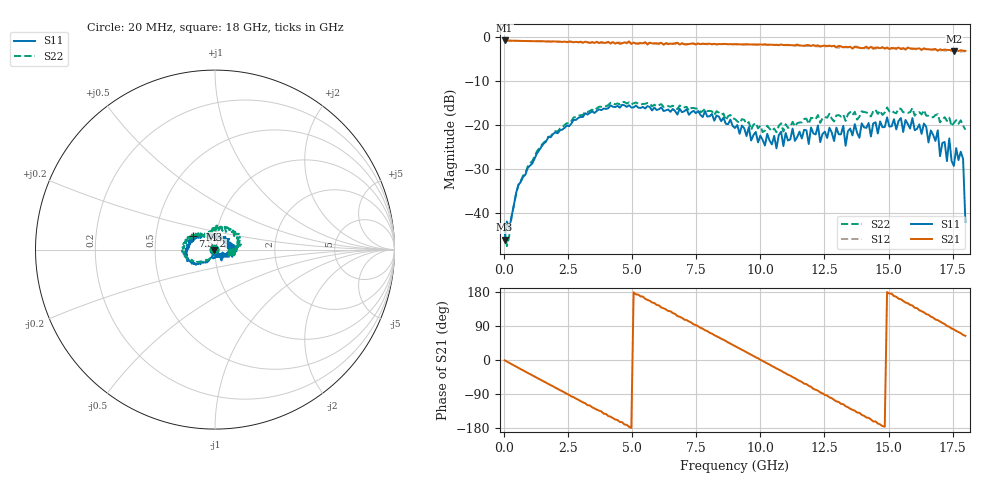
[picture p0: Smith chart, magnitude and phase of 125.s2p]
!Agilent Technologies,N5230A,US43500223,A.07.50.48
!Agilent N5230A: A.07.50.48
!Date: Sunday, January 31, 2016 17:07:24
!Correction: S11(Full 2 Port(1,2))
!S21(Full 2 Port(1,2))
!S12(Full 2 Port(1,2))
!S22(Full 2 Port(1,2))
!S2P File: Measurements: S11, S21, S12, S22:
# Hz S  RI  R 50
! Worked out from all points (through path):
!   201 points, 20 MHz to 18 GHz, reference 50 ohm
!   highest |S21| = -0.70 dB at 20 MHz (marker M1); lowest = -3.1 dB at 17.55 GHz (marker M2)
!   group delay of S21, straight-line fit = 101 ps
!   lowest |S11| = -46.1 dB at 20 MHz (marker M3), VSWR 1.01, Z = 49.5 + j0.051 ohm
!   |S11| at or under -10 dB: start of sweep to end of sweep
!   |S22| runs from -47.6 to -14.7 dB; largest |S21 - S12| = 0.07
!   S11 on the Smith chart (normalised r, x): 20 MHz: 0.99, +0.00; 7.572 GHz: 0.77, +0.12; 18 GHz: 1.00, -0.02
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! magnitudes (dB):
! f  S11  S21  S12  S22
! 20 MHz  -46.1  -0.7  -0.7  -44.0
! 109.9 MHz  -41.9  -0.7  -0.7  -47.6
! 559.4 MHz  -33.6  -0.8  -0.8  -33.6
! 1.279 GHz  -26.4  -0.9  -0.9  -26.0
! 3.077 GHz  -18.1  -1.2  -1.1  -17.7
! 6.043 GHz  -16.4  -1.4  -1.6  -15.4
! 7.572 GHz  -16.8  -1.4  -1.3  -16.2
! 9.01 GHz  -20.6  -1.5  -1.5  -18.6
! 10.63 GHz  -25.3  -1.7  -1.7  -21.6
! 12.07 GHz  -21.9  -1.7  -1.9  -18.4
! 13.24 GHz  -20.1  -2.3  -2.2  -17.6
! 13.33 GHz  -24.7  -2.1  -2.2  -19.0
! 15.03 GHz  -20.3  -2.7  -2.6  -16.9
! 16.92 GHz  -21.2  -3.0  -3.0  -17.5
! 17.01 GHz  -27.1  -2.7  -3.0  -19.3
! 17.19 GHz  -23.8  -2.8  -3.0  -18.2
! 17.28 GHz  -28.2  -2.9  -3.0  -19.0
! 17.37 GHz  -23.0  -2.9  -3.1  -18.3
! 17.55 GHz  -29.3  -3.1  -3.2  -19.5
! 17.64 GHz  -25.2  -2.9  -3.1  -18.9
! 17.91 GHz  -27.7  -3.0  -3.1  -20.1
! 18 GHz  -42.0  -3.1  -3.3  -21.0
